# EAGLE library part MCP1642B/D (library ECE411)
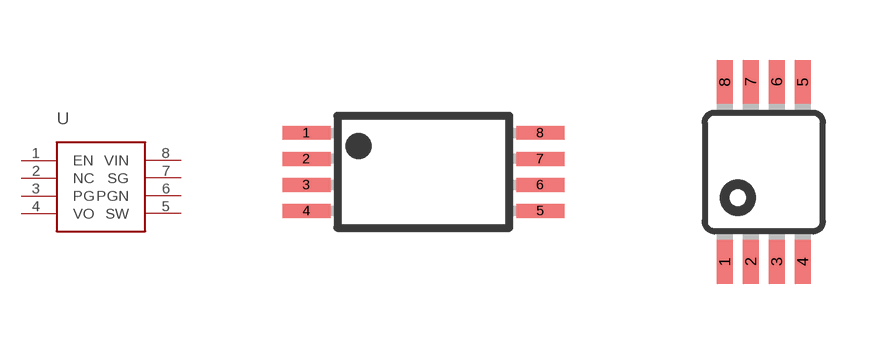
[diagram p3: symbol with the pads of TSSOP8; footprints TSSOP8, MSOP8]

Designator prefix -

## MCP1642B/D  [TSSOP8]
1  EN
2  NC
3  PG
4  VO
5  SW
6  PGN
7  SG
8  VIN

## MCP1642B/D8-MSOP  [MSOP8]
Pads as for TSSOP8

## Footprint TSSOP8 (pad centres in mm)
8-Pin Molded TSSOP, JEDEC (MT8) Package Number MTC08 Source: www.fairchildsemi.com
smd 1.2 x 0.35: 1 -2.925,0.975; 2 -2.925,0.325; 3 -2.925,-0.325; 4 -2.925,-0.975; 5 2.925,-0.975; 6 2.925,-0.325; 7 2.925,0.325; 8 2.925,0.975

## Footprint MSOP8 (pad centres in mm)
8M, 8-Lead, 0.118" Wide, Miniature Small Outline Package MSOP 8M-Package doc1097.pdf
smd 0.4 x 1.1: 1 -0.975,-2.25; 2 -0.325,-2.25; 3 0.325,-2.25; 4 0.975,-2.25; 5 0.975,2.25; 6 0.325,2.25; 7 -0.325,2.25; 8 -0.975,2.25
